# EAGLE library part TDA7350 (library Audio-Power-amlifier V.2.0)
The TDA7350 22W BRIDGE-STEREO AMPLIFIER FOR CAR RADIO,is a new technology class AB Audio Power Amplifier in the Multiwatt® package designed for car radio applications
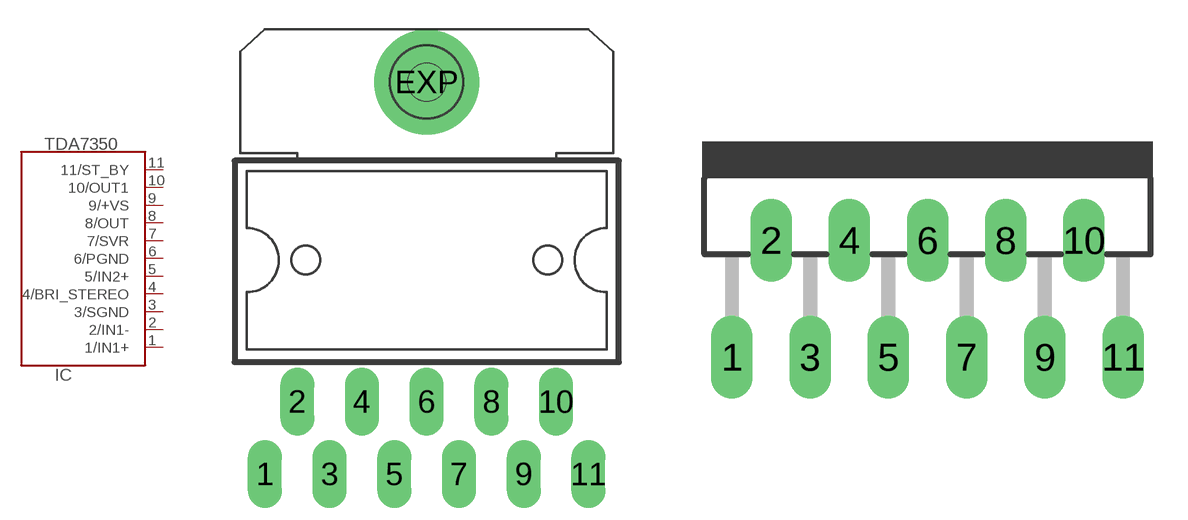
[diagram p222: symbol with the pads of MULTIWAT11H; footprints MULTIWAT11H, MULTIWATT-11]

Designator prefix IC

## TDA7350H  [MULTIWAT11H]
1  1/IN1+  in
2  2/IN1-  in
3  3/SGND  pwr
4  4/BRI_STEREO  in
5  5/IN2+  in
6  6/PGND  pwr
7  7/SVR
8  8/OUT  out
9  9/+VS  pwr
10  10/OUT1  out
11  11/ST_BY  in

## TDA7350V  [MULTIWATT-11]
Pads as for MULTIWAT11H

## Footprint MULTIWAT11H (pad centres in mm)
Multiwatt11 H (Short leads)
drill 0.9 pad 1.778 long: 1 -8.5,-3.81; 2 -6.8,0; 3 -5.1,-3.81; 4 -3.4,0; 5 -1.7,-3.81; 6 0,0; 7 1.7,-3.81; 8 3.4,0; 9 5.1,-3.81; 10 6.8,0; 11 8.5,-3.81
drill 3.2 pad 5.5: EXP 0,16.81
hole 2 at 0,16.81

## Footprint MULTIWATT-11 (pad centres in mm)
Muliwatt 11 lead
drill 1.2 long: 1 -8.5,-6.35; 2 -6.8,-1.27; 3 -5.1,-6.35; 4 -3.4,-1.27; 5 -1.7,-6.35; 6 0,-1.27; 7 1.7,-6.35; 8 3.4,-1.27; 9 5.1,-6.35; 10 6.8,-1.27; 11 8.5,-6.35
